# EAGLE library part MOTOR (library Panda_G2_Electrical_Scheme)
Motor
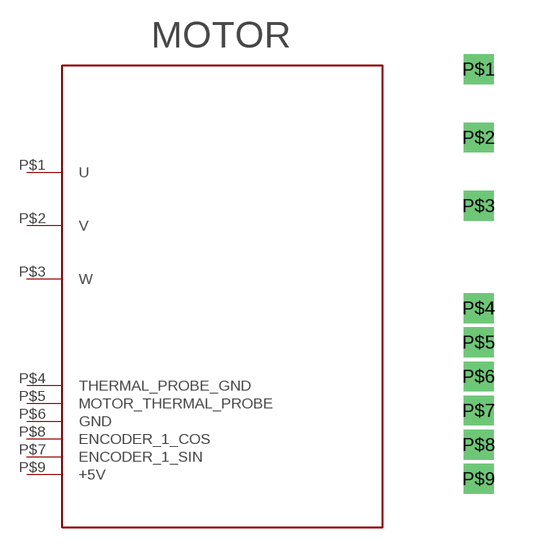
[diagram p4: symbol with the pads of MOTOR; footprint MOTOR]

Designator prefix -

## MOTOR  [MOTOR]
P$1  U
P$2  V
P$3  W
P$4  THERMAL_PROBE_GND
P$5  MOTOR_THERMAL_PROBE
P$6  GND
P$7  ENCODER_1_SIN
P$8  ENCODER_1_COS
P$9  +5V

## Footprint MOTOR (pad centres in mm)
drill 0.6 square: P$1 -1.27,24.13; P$2 -1.27,21.59; P$3 -1.27,19.05; P$4 -1.27,15.24; P$5 -1.27,13.97; P$6 -1.27,12.7; P$7 -1.27,11.43; P$8 -1.27,10.16; P$9 -1.27,8.89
